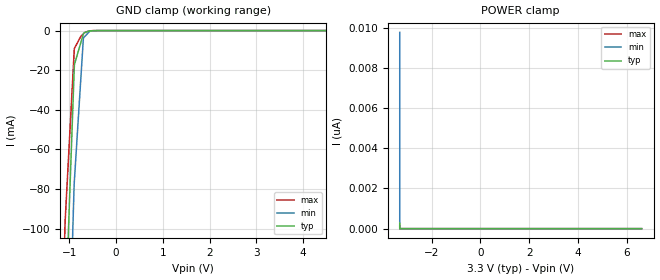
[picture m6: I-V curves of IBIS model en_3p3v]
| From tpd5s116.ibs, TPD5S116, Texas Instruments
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[Model]   en_3p3v
Model_type   Input
Vinl = 0.4
Vinh = 1
|   typ   min   max
|   (nom PVT)   (slow PVT)   (fast PVT)
C_comp   0.787p   0.739p   0.858p
| Where nom  PVT is Nominal Process, 3.3V, 27C
|   Fast PVT is Strong Process,  3.6V, -40C
|   Slow PVT is Weak Process,   3.0V, 125C
[Voltage Range]   3.3   3   3.6
[Temperature Range]   27   125   -40
[Power Clamp Reference]   3.3   3   3.6
[GND Clamp Reference]   -0   -0   -0
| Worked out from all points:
|   GND clamp passes 1 mA (typ) near -0.67 V on its own axis
[GND Clamp]
|   Voltage   I(typ)   I(min)   I(max)
-3.3V     -2.279A    -2.354A    -2.233A
-1.291V   -323.3mA   -408.2mA   -269.8mA
-1.098V   -151.8mA   -235.1mA   -100.1mA
-1.093V   -147.3mA   -231.1mA   -96.22mA
-900.1mV  -20.53mA   -77.67mA   -10.72mA
-896.5mV  -18.11mA   -76.3mA    -9.094mA
-755.1mV  -5.933mA   -23.5mA    -2.819mA
-702.1mV  -1.668mA   -3.733mA   -1.641mA
-666.7mV  -974.7uA   -2.86mA    -853.9uA
-564.7mV  -200.7uA   -342.6uA   -132uA
-427.3mV  -16.17uA   -32.17uA   -6.936uA
6.6V      0A         0A         0A
[POWER Clamp]
|   Voltage   I(typ)   I(min)   I(max)
-3.3V     270.8pA    9.769nA    124.7pA
-3.3V     0A         0A         0A
-3.3V     0A         0A         0A
6.6V      0A         0A         0A
